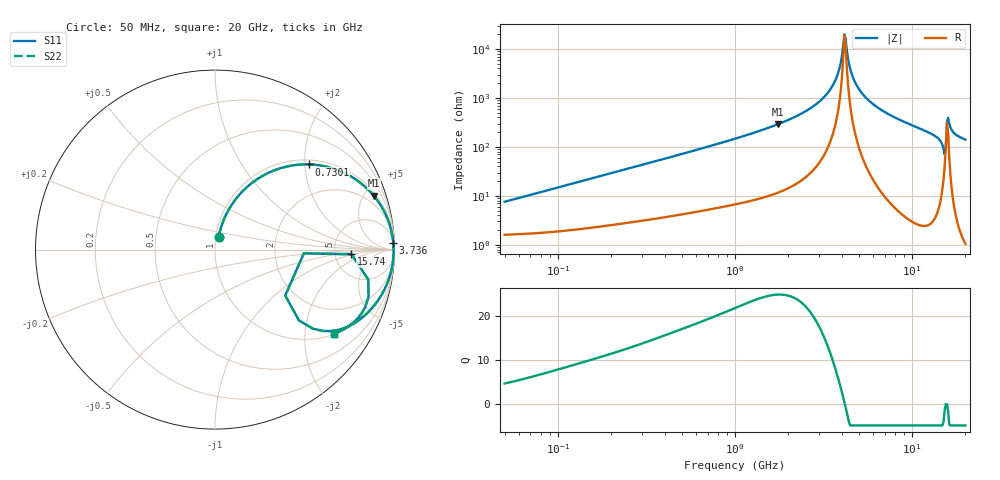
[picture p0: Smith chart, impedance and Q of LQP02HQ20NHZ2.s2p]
!Murata Part Number: LQP02HQ20NHZ2
!These Parameters are Measured in Series Mode Connection
!  o--[Z]--o
!Port1  Port2
!  o-------o
!Freq. Start=50[MHz] Stop=20[GHz], 401[Steps]
# Hz S RI R 50
!Freq.(Hz) S11(Real) S11(Imag) S21(Real) S21(Imag) S12(Real) S12(Imag) S22(Real) S22(Imag)
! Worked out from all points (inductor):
!   401 points, 50 MHz to 20 GHz, reference 50 ohm
!   read as one part in series: L = 23.5 nH near 51.52 MHz
!   highest Q = 25 at 1.741 GHz (marker M1), where L = 26.4 nH
!   self-resonance near 4.149 GHz
!   S11 on the Smith chart (normalised r, x): 50 MHz: 1.03, +0.15; 730.1 MHz: 1.11, +2.10; 3.736 GHz: 8, +51; 15.74 GHz: 7.23, -0.89; 20 GHz: 1.02, -2.81
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5e7  0.021 0.0714  0.979 -0.0714  0.979 -0.0714  0.021 0.0714
1.364002e8  0.0567 0.1842  0.9433 -0.1842  0.9433 -0.1842  0.0567 0.1842
3.721004e8  0.2357 0.3928  0.7643 -0.3928  0.7643 -0.3928  0.2357 0.3928
7.30116e8  0.5235 0.4747  0.4765 -0.4747  0.4765 -0.4747  0.5235 0.4747
1e9  0.6759 0.4458  0.3241 -0.4458  0.3241 -0.4458  0.6759 0.4458
1.740566e9  0.8836 0.3014  0.1164 -0.3014  0.1164 -0.3014  0.8836 0.3014
2.728004e9  0.97 0.1478  0.03 -0.1478  0.03 -0.1478  0.97 0.1478
3.314454e9  0.9876 0.0799  0.0124 -0.0799  0.0124 -0.0799  0.9876 0.0799
3.736399e9  0.9932 0.0381  0.00676 -0.0381  0.00676 -0.0381  0.9932 0.0381
4.087748e9  0.9951 0.00667  0.00493 -0.00667  0.00493 -0.00667  0.9951 0.00667
4.212059e9  0.9952 -0.00381  0.00478 0.00381  0.00478 0.00381  0.9952 -0.00381
4.539627e9  0.9946 -0.0301  0.0054 0.0301  0.0054 0.0301  0.9946 -0.0301
4.966507e9  0.9919 -0.0618  0.00806 0.0618  0.00806 0.0618  0.9919 -0.0618
5.856089e9  0.9814 -0.1205  0.0186 0.1205  0.0186 0.1205  0.9814 -0.1205
7.442007e9  0.951 -0.2078  0.049 0.2078  0.049 0.2078  0.951 -0.2078
1.183995e10  0.8163 -0.3816  0.1837 0.3816  0.1837 0.3816  0.8163 -0.3816
1.438523e10  0.64 -0.4542  0.36 0.4542  0.36 0.4542  0.64 -0.4542
1.504638e10  0.4678 -0.3947  0.5322 0.3947  0.5322 0.3947  0.4678 -0.3947
1.573793e10  0.7599 -0.0259  0.2401 0.0259  0.2401 0.0259  0.7599 -0.0259
1.646126e10  0.8376 -0.3188  0.1624 0.3188  0.1624 0.3188  0.8376 -0.3188
1.747767e10  0.7665 -0.4105  0.2335 0.4105  0.2335 0.4105  0.7665 -0.4105
2e10  0.6632 -0.4689  0.3368 0.4689  0.3368 0.4689  0.6632 -0.4689
